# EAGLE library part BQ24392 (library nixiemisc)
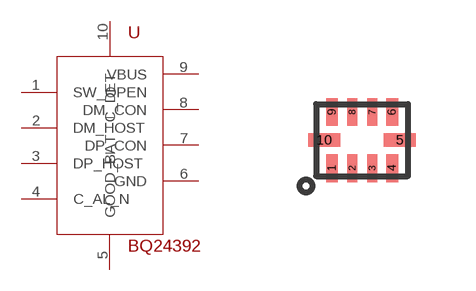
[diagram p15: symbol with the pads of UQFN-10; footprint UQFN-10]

Designator prefix -

## BQ24392  [UQFN-10]
1  SW_OPEN  pas
2  DM_HOST  pas
3  DP_HOST  pas
4  C_AL_N  pas
5  GOOD_BAT  pas
6  GND  pwr
7  DP_CON  pas
8  DM_CON  pas
9  VBUS  pwr
10  C_DET  pas

## Footprint UQFN-10 (pad centres in mm)
smd 0.3 x 0.7: 1 -0.75,-0.7; 4 0.75,-0.7; 6 0.75,0.7; 9 -0.75,0.7
smd 0.25 x 0.7: 2 -0.25,-0.7; 3 0.25,-0.7; 7 0.25,0.7; 8 -0.25,0.7
smd 0.8 x 0.35: 5 0.945,0; 10 -0.945,0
